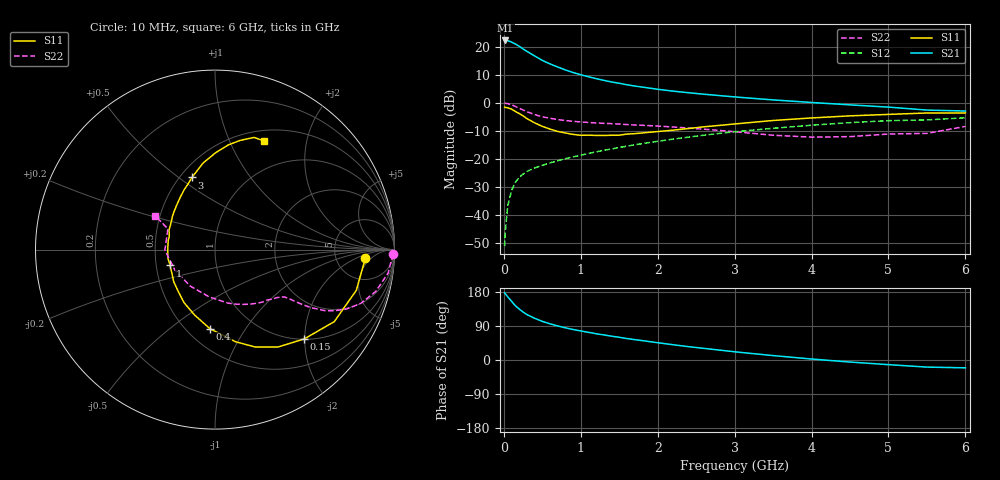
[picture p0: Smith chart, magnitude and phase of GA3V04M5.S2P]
! Infineon Technologies  Discrete & RF Semiconductors
! BF775
! Si NPN RF Bipolar Junction Transistor in SOT23
! VCE = 3 V  IC = 4.5 mA
! Common Emitter S-Parameters:  May  1996
# GHz  S  MA  R  50
!  f  S11  S21  S12  S22
! GHz  MAG  ANG  MAG  ANG  MAG  ANG  MAG  ANG
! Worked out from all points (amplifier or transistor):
!   36 points, 10 MHz to 6 GHz, reference 50 ohm
!   highest |S21| = 22.3 dB at 20 MHz (marker M1)
!   |S21| within 3 dB of that: start of sweep to 248.1 MHz
!   unconditionally stable (mu >= 1): 830 MHz to 3.523 GHz
!   at 250 MHz: K = 0.46, MSG = 22.3 dB, |S12| = -25.4 dB
!   at 1.4 GHz: K = 1.13, MAG = 9.7 dB, |S12| = -16.4 dB
!   at 6 GHz: K = 0.97, MSG = 1.2 dB, |S12| = -5.3 dB
!   S11 on the Smith chart (normalised r, x): 10 MHz: 10, -3; 150 MHz: 1.01, -1.99; 400 MHz: 0.64, -0.71; 1 GHz: 0.59, -0.11; 3 GHz: 0.57, +0.56; 6 GHz: 0.63, +1.36
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0.01  0.8395 -3.3  12.95 177.4  0.0028 86.5  0.993 -1.5
0.02  0.831 -6.2  12.99 174.4  0.0053 84.8  0.9859 -3.1
0.05  0.8193 -16.1  12.94 166.9  0.0145 81.1  0.9726 -7.8
0.1  0.7765 -31.1  12.13 155.0  0.0273 74.4  0.9263 -14.5
0.15  0.7037 -45.0  11.25 143.1  0.0386 67.6  0.8666 -20.2
0.2  0.6468 -57.0  10.21 134.4  0.0471 63.3  0.8042 -24.3
0.25  0.5875 -67.5  9.156 126.6  0.054 59.5  0.748 -27.1
0.3  0.5262 -77.4  8.31 119.9  0.0601 57.6  0.699 -29.1
0.4  0.4418 -93.6  6.878 110.1  0.0693 55.5  0.6197 -31.3
0.5  0.3824 -107.2  5.727 101.9  0.0772 54.1  0.5663 -32.3
0.6  0.3422 -120.3  4.96 95.5  0.0855 54.0  0.5335 -32.9
0.8  0.2914 -142.1  3.877 84.9  0.1014 54.7  0.4858 -33.8
1  0.2652 -160.5  3.181 76.7  0.1171 55.5  0.458 -35.1
1.1  0.2663 -169.2  2.932 73.0  0.1255 55.7  0.4491 -36.2
1.3  0.2632 175.8  2.521 66.1  0.143 55.6  0.4328 -38.4
1.6  0.2789 156.7  2.109 56.6  0.1698 54.9  0.4117 -42.6
2.2  0.3272 130.7  1.622 40.3  0.2266 51.8  0.3723 -53.9
3  0.4221 107.7  1.28 21.7  0.3059 44.3  0.3069 -76.3
3.5  0.4866 97.9  1.132 11.6  0.3536 38.4  0.2656 -96.9
4.5  0.5884 82.7  0.924 -5.4  0.4455 25.6  0.251 -153.3
5.5  0.6618 70.8  0.746 -18.7  0.4979 10.6  0.2867 156.2
6  0.6639 65.6  0.717 -20.7  0.5434 6.4  0.3814 150.6
